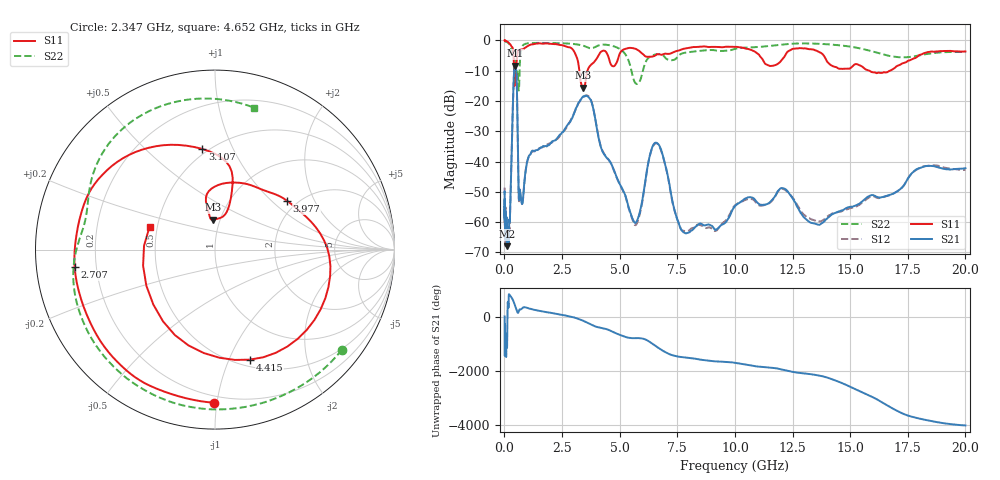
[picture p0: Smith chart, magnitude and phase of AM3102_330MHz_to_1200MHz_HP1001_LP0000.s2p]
! Date/Time: Tue, Sep 11, 2018 5:17 PM
! Network Analyzer: Agilent Technologies E8362B Rev: A.07.50.63
! Sweep from 0.010 to 20.000 GHz, 1601 Points, Sweep Type: LOG
! Power Supply: 4.949 V, 0.001 A
# Hz S DB R 50
!freq MagS11 AngS11 MagS21 AngS21 MagS12 AngS12 MagS22 AngS22
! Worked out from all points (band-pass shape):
!   1601 points, 10 MHz to 20 GHz, reference 50 ohm
!   highest |S21| = -8.35 dB at 458 MHz (marker M1); lowest = -67.9 dB at 126.4 MHz (marker M2)
!   |S21| within 3 dB of the highest: 413.6 MHz to 525.1 MHz (111.4 MHz wide, 23.7 % of centre)
!   lowest |S11| = -15.6 dB at 3.432 GHz (marker M3), VSWR 1.40, Z = 46.3 + j15.9 ohm
!   |S11| at or under -10 dB: 419 MHz to 466.4 MHz (47.48 MHz wide, 10.7 % of centre); 3.251 GHz to 3.604 GHz (353.1 MHz wide, 10.3 % of centre); 15.84 GHz to 16.72 GHz (879.5 MHz wide, 5.4 % of centre)
!   |S22| runs from -16.5 to -0.2 dB; largest |S21 - S12| = 0.0049
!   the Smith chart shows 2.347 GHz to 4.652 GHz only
!   S11 on the Smith chart (normalised r, x): 2.347 GHz: 0.16, -0.98; 2.707 GHz: 0.12, -0.06; 3.107 GHz: 0.47, +0.77; 3.977 GHz: 1.77, +1.26; 4.415 GHz: 0.57, -1.19; 4.652 GHz: 0.45, +0.13
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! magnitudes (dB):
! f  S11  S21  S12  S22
! 10 MHz  0.0  -50.0  -48.6  -0.2
! 35.55 MHz  0.0  -64.1  -63.7  -0.2
! 126.4 MHz  -0.4  -67.9  -63.9  -0.6
! 237.7 MHz  -1.2  -59.4  -58.8  -1.5
! 447.2 MHz  -14.7  -8.5  -8.5  -6.4
! 458 MHz  -12.3  -8.3  -8.4  -6.5
! 533.2 MHz  -7.2  -13.0  -13.0  -12.1
! 632.6 MHz  -3.2  -52.5  -53.0  -16.2
! 757.7 MHz  -2.9  -53.9  -53.9  -2.3
! 1.59 GHz  -1.0  -35.3  -35.3  -0.8
! 2.347 GHz  -1.4  -31.7  -32.1  -0.9
! 2.707 GHz  -2.1  -28.3  -28.7  -1.0
! 3.107 GHz  -5.0  -22.3  -22.5  -1.3
! 3.432 GHz  -15.6  -18.5  -18.6  -1.8
! 3.977 GHz  -6.3  -27.5  -27.3  -2.0
! 4.415 GHz  -3.8  -38.5  -38.4  -1.4
! 4.652 GHz  -8.3  -41.0  -41.1  -1.7
! 5.652 GHz  -2.6  -60.1  -60.9  -13.7
! 6.549 GHz  -4.9  -33.8  -34.0  -4.6
! 7.92 GHz  -2.5  -63.6  -62.9  -3.9
! 13.68 GHz  -3.9  -60.9  -59.7  -1.1
! 20 GHz  -3.6  -42.2  -42.8  -3.8
